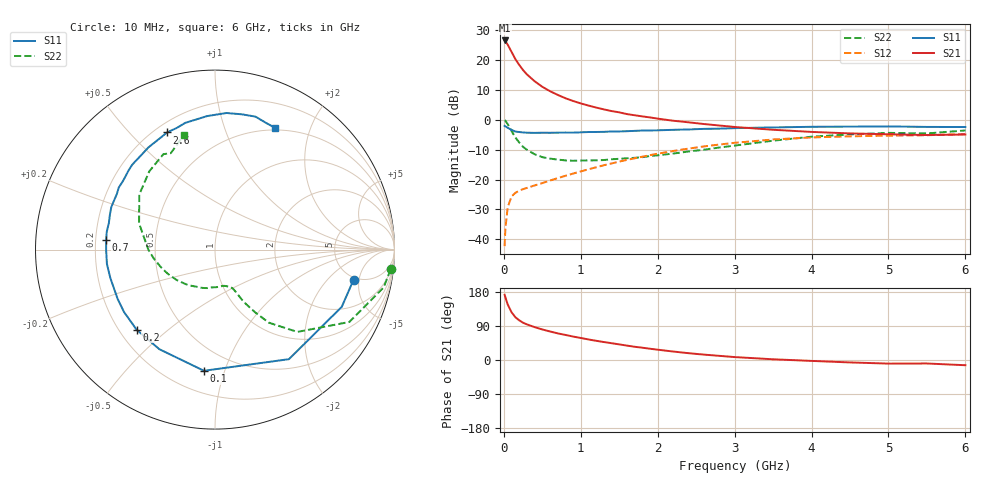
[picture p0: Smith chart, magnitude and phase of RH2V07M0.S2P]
! SIEMENS Small Signal Semiconductors
! BFR106
! Si NPN RF Bipolar Junction Transistor in SOT23
! VCE = 2 V  IC = 7 mA
! Common Emitter S-Parameters:  August  1996
# GHz  S  MA  R  50
!  f  S11  S21  S12  S22
! GHz  MAG  ANG  MAG  ANG  MAG  ANG  MAG  ANG
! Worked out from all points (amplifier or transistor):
!   36 points, 10 MHz to 6 GHz, reference 50 ohm
!   highest |S21| = 26.5 dB at 10 MHz (marker M1)
!   |S21| within 3 dB of that: start of sweep to 83.24 MHz
!   unconditionally stable (mu >= 1): 540 MHz to 2.28 GHz; 4.478 GHz to end of sweep
!   at 250 MHz: K = 0.61, MSG = 19.9 dB, |S12| = -23.2 dB
!   at 1.4 GHz: K = 1.13, MAG = 6.5 dB, |S12| = -14.6 dB
!   at 6 GHz: K = 1.03, MAG = -1.1 dB, |S12| = -4.8 dB
!   S11 on the Smith chart (normalised r, x): 10 MHz: 4.68, -4.19; 100 MHz: 0.34, -0.85; 200 MHz: 0.27, -0.39; 700 MHz: 0.24, +0.04; 2.6 GHz: 0.25, +0.64; 6 GHz: 0.47, +1.50
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0.01  0.7901 -12.3  21.22 172.0  0.0077 84.5  0.9848 -6.4
0.02  0.7749 -24.3  20.64 165.6  0.0151 78.6  0.9633 -12.6
0.05  0.7364 -56.0  18.05 146.6  0.0342 63.3  0.8504 -28.3
0.1  0.6779 -95.2  13.7 126.1  0.0523 48.7  0.6486 -45.0
0.15  0.6357 -119.2  10.33 112.8  0.06 42.2  0.5059 -53.6
0.2  0.6243 -134.4  8.279 104.7  0.0651 39.9  0.4169 -57.3
0.25  0.6147 -145.5  6.781 98.3  0.0692 39.3  0.3521 -60.2
0.3  0.608 -153.2  5.747 94.0  0.0725 40.1  0.3157 -61.8
0.4  0.6043 -165.0  4.412 86.7  0.0798 42.7  0.2652 -63.7
0.5  0.6074 -172.5  3.565 80.6  0.0873 45.5  0.2372 -65.5
0.6  0.6064 -179.4  3.008 75.3  0.0964 48.2  0.2242 -68.0
0.7  0.6088 174.9  2.61 70.3  0.1057 50.5  0.2162 -71.3
0.9  0.6096 165.9  2.064 61.9  0.1261 53.7  0.2066 -77.8
1.1  0.6243 157.8  1.729 54.2  0.1485 55.8  0.2093 -87.2
1.3  0.6287 150.3  1.493 47.4  0.1736 56.6  0.2123 -96.2
1.6  0.6443 140.7  1.246 38.0  0.2135 56.2  0.2275 -111.2
2.2  0.6796 123.1  0.965 22.4  0.3005 50.6  0.2724 -141.5
2.6  0.7052 112.2  0.85 14.2  0.3582 44.8  0.3158 -161.6
3.5  0.7451 93.4  0.681 1.9  0.4687 29.3  0.4473 161.0
4.5  0.7684 78.8  0.592 -6.4  0.5291 12.1  0.5694 130.0
5.5  0.7602 67.6  0.556 -9.2  0.5519 1.7  0.591 114.6
6  0.7565 63.8  0.567 -13.8  0.577 -5.6  0.6635 105.0
